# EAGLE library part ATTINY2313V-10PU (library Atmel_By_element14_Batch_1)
Microcontroller
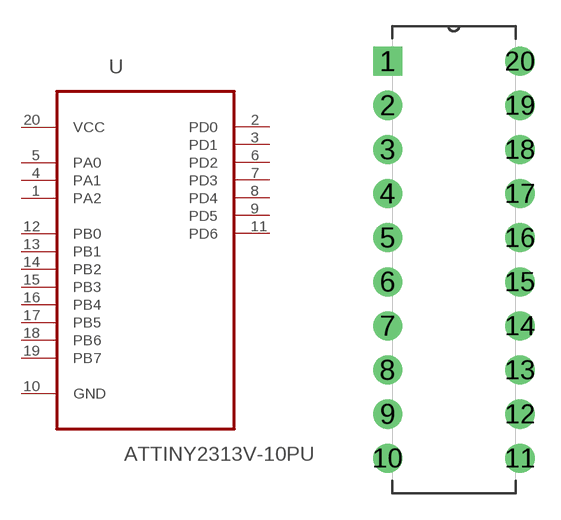
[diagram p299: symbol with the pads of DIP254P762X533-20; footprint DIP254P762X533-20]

Designator prefix U

## ATTINY2313V-10PU (MPN: ATTINY2313V-10PU; OC_FARNELL: 9171614; OC_NEWARK: 01M6916; PACKAGE: DIP-20; SUPPLIER: ATMEL)  [DIP254P762X533-20]
1  PA2
2  PD0
3  PD1
4  PA1
5  PA0
6  PD2
7  PD3
8  PD4
9  PD5
10  GND  pas
11  PD6
12  PB0
13  PB1
14  PB2
15  PB3
16  PB4
17  PB5
18  PB6
19  PB7
20  VCC  pwr

## Footprint DIP254P762X533-20 (pad centres in mm)
drill 1.118 square: 1 -7.62,22.86
drill 1.118: 2 -7.62,20.32; 3 -7.62,17.78; 4 -7.62,15.24; 5 -7.62,12.7; 6 -7.62,10.16; 7 -7.62,7.62; 8 -7.62,5.08; 9 -7.62,2.54; 10 -7.62,0; 11 0,0; 12 0,2.54; 13 0,5.08; 14 0,7.62; 15 0,10.16; 16 0,12.7; 17 0,15.24; 18 0,17.78; 19 0,20.32; 20 0,22.86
